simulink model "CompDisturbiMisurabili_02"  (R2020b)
settings: Solver=FixedStepAuto  StartTime=0.0  StopTime=400  FixedStep=0.01  RelTol=1e-3  EnableMultiTasking=on
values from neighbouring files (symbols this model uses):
  delta1 = 14.7    [CompDisturbiMisurabili_02_script.m]
  delta2 = 13    [CompDisturbiMisurabili_02_script.m]
  deltaf = max((delta2-delta1),0)    [CompDisturbiMisurabili_02_script.m]
  k1 = 1    [CompDisturbiMisurabili_02_script.m]
  k2 = 1    [CompDisturbiMisurabili_02_script.m]
  T1 = 21.3    [CompDisturbiMisurabili_02_script.m]
  T2 = 25    [CompDisturbiMisurabili_02_script.m]

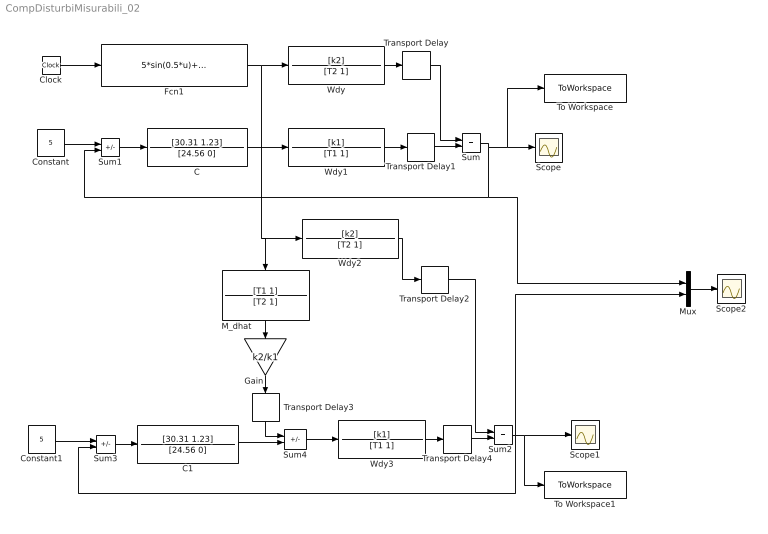
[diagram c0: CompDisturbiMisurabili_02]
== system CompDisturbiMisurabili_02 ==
  C : TransferFcn  Numerator=[30.31 1.23]  Denominator=[24.56 0]
  C1 : TransferFcn  Numerator=[30.31 1.23]  Denominator=[24.56 0]
  Clock : Clock
  Constant : Constant  Value=5
  Constant1 : Constant  Value=5
  Fcn1 : Fcn  Expr=5*sin(0.5*u)+cos(u)
  Gain : Gain  Gain=k2/k1
  "M_dhat " : TransferFcn  Numerator=[T1 1]  Denominator=[T2 1]
  Mux : Mux  Inputs=2
  Scope : Scope
  Scope1 : Scope
  Scope2 : Scope
  Sum : Sum
  Sum1 : Sum  Inputs=+-
  Sum2 : Sum
  Sum3 : Sum  Inputs=+-
  Sum4 : Sum  Inputs=-+
  To Workspace : ToWorkspace  VariableName=y  SaveFormat=Timeseries  SampleTime=-1
  To Workspace1 : ToWorkspace  VariableName=y_comp  SaveFormat=Timeseries  SampleTime=-1
  Transport Delay : TransportDelay  DelayTime=delta2  BufferSize=10000
  Transport Delay1 : TransportDelay  DelayTime=delta1  BufferSize=10000
  Transport Delay2 : TransportDelay  DelayTime=delta2  BufferSize=10000
  Transport Delay3 : TransportDelay  DelayTime=deltaf  BufferSize=10000
  Transport Delay4 : TransportDelay  DelayTime=delta1  BufferSize=10000
  Wdy : TransferFcn  Numerator=[k2]  Denominator=[T2 1]
  Wdy1 : TransferFcn  Numerator=[k1]  Denominator=[T1 1]
  Wdy2 : TransferFcn  Numerator=[k2]  Denominator=[T2 1]
  Wdy3 : TransferFcn  Numerator=[k1]  Denominator=[T1 1]
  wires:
  C/1 -> Wdy1/1
  Sum1/1 -> C/1
  Sum/1 -> To Workspace/1, Scope/1, Mux/1, Sum1/2
  Sum3/1 -> C1/1
  Sum2/1 -> Mux/2, Sum3/2, To Workspace1/1, Scope1/1
  Constant/1 -> Sum1/1
  C1/1 -> Sum4/2
  Sum4/1 -> Wdy3/1
  Mux/1 -> Scope2/1
  Wdy/1 -> Transport Delay/1
  Wdy1/1 -> Transport Delay1/1
  Constant1/1 -> Sum3/1
  Fcn1/1 -> Wdy/1, "M_dhat "/1, Wdy2/1
  Clock/1 -> Fcn1/1
  Transport Delay/1 -> Sum/1
  Transport Delay1/1 -> Sum/2
  Wdy2/1 -> Transport Delay2/1
  Transport Delay2/1 -> Sum2/1
  Transport Delay3/1 -> Sum4/1
  Transport Delay4/1 -> Sum2/2
  Wdy3/1 -> Transport Delay4/1
  Gain/1 -> Transport Delay3/1
  "M_dhat "/1 -> Gain/1
